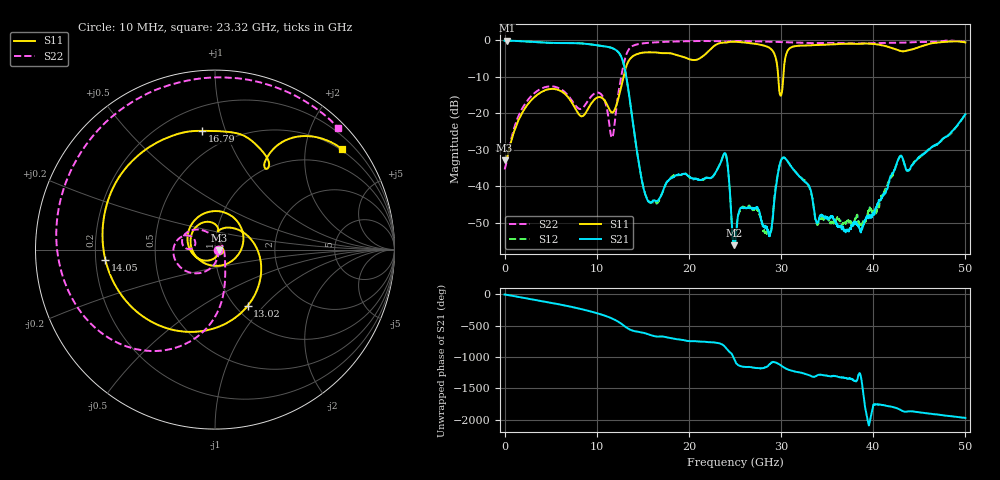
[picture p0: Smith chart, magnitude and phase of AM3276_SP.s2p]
!Keysight Technologies,N5245B,MY58422270,A.16.20.02
!Date: Friday, January 23, 2026 00:46:15
!Correction: S11(C  2-Port  )
!S21(C  2-Port  )
!S12(C  2-Port  )
!S22(C  2-Port  )
!S2P File: Measurements: S11, S21, S12, S22:
# Hz S  dB  R 50
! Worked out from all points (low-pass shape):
!   3201 points, 10 MHz to 50 GHz, reference 50 ohm
!   highest |S21| = -0.19 dB at 275.6 MHz (marker M1); lowest = -56.0 dB at 24.93 GHz (marker M2)
!   |S21| within 3 dB of the highest: start of sweep to 12.3 GHz
!   lowest |S11| = -32.9 dB at 10 MHz (marker M3), VSWR 1.05, Z = 52.3 - j0.478 ohm
!   |S11| at or under -10 dB: start of sweep to 12.91 GHz; 29.69 GHz to 30.24 GHz (550 MHz wide, 1.84 % of centre)
!   |S22| runs from -35.3 to -0.1 dB; largest |S21 - S12| = 0.011
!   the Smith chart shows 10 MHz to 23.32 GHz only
!   S11 on the Smith chart (normalised r, x): 10 MHz: 1.05, -0.01; 13.02 GHz: 1.13, -0.82; 14.05 GHz: 0.24, -0.05; 16.79 GHz: 0.35, +0.83; 23.32 GHz: 0.46, +2.79
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1e7  -32.88 -11.6  -0.22 -2.4  -0.17 -1.8  -35.35 -7.6
2.755719e8  -32.18 -37.5  -0.19 -7.5  -0.18 -7.4  -32.55 -36.5
3.868603e9  -14.42 134.5  -0.67 -102.5  -0.65 -102.5  -13.44 -150.4
8.352081e9  -20.85 -94.0  -0.95 124.4  -0.95 124.3  -18.78 169.3
1.11484e10  -17.76 84.6  -1.87 6.5  -1.87 6.4  -19.28 114.8
1.225755e10  -16.80 58.1  -3.10 -68.9  -3.10 -68.9  -16.13 -68.6
1.302302e10  -8.81 -59.9  -7.62 -147.5  -7.62 -147.6  -5.59 -104.7
1.405407e10  -4.25 -174.5  -24.98 134.9  -24.96 135.1  -1.47 -162.5
1.667854e10  -3.50 98.2  -43.76 46.7  -44.18 48.6  -0.60 133.3
1.678789e10  -3.54 96.3  -43.44 47.3  -43.72 47.4  -0.59 131.5
2.331784e10  -0.89 38.5  -34.24 -61.9  -34.17 -62.8  -0.32 44.5
2.408331e10  -0.71 25.3  -31.97 -146.9  -32.03 -147.5  -0.48 36.4
2.492689e10  -0.49 11.4  -56.03 47.1  -56.10 35.8  -0.29 26.7
2.5005e10  -0.49 10.1  -55.47 21.8  -55.85 9.6  -0.28 25.7
2.894171e10  -2.55 -64.1  -52.07 -8.9  -51.69 148.1  -0.48 -20.4
3.022271e10  -10.81 34.4  -32.08 -78.7  -32.14 -79.9  -0.57 -35.6
3.334708e10  -1.45 -92.4  -42.51 129.8  -42.68 134.0  -0.86 -72.3
3.761185e10  -1.02 169.6  -50.84 92.2  -50.38 85.7  -0.94 -122.9
4.167354e10  -1.94 44.5  -39.14 15.0  -38.83 14.1  -0.79 -167.8
4.434488e10  -2.50 -98.8  -33.77 -69.3  -33.70 -69.9  -0.62 165.2
4.643821e10  -0.89 -177.3  -29.04 -110.2  -29.17 -112.1  -0.54 144.5
5e10  -0.69 120.4  -20.29 -171.5  -20.63 -170.4  -0.55 109.0
